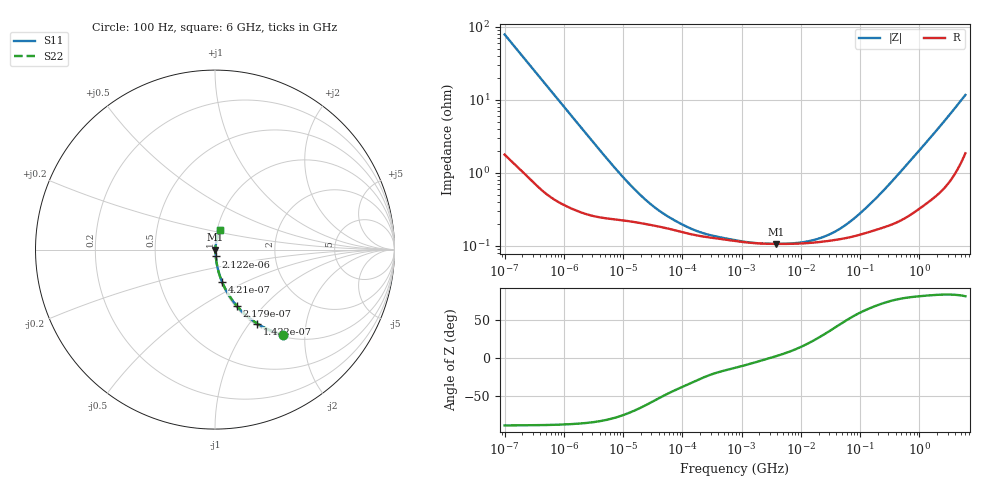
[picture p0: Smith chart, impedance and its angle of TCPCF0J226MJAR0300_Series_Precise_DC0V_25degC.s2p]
! TCPCF0J226MJAR0300 Polymer Tantalum Capacitor Sparameter Model
! Model Generated by Samsung Electro-Mechanics
! Samsung Sparameter Version 5.0
! Date : Oct-10-2024
! Products : Polymer Tantalum Capacitor
! Characteristics :
!  Nominal Capacitance = 22uF
!  Capacitance Tolerance = +/-20%
!  ESR = 300 mohm max at 100kHz
!  Rated Voltage = 6.3Vdc
!  Size = 0603(unit:inch), 1608(unit:mm)
!  Length = 1.60+/-0.20mm
!  Width = 0.80+/-0.20mm
!  Thickness = 0.90+/-0.10mm
!  Lineup = Conductive Polymer Type
!  Feature = PCF
!  Measurement Temperature : 25degC.
!  DC bias Value = 0V
!  Frequency : 100Hz ~ 6GHz
! External Node Assignments :
!  1  o---||---o  2
# MHz S RI R 50.0
! Freq.  Real(S11)  Im(S11)  Real(S12)  Im(S12)  Real(S21)  Im(S21)  Real(S22)  Im(S22)
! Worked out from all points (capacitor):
!   300 points, 100 Hz to 6 GHz, reference 50 ohm
!   read as one part in series: C = 20.4 uF near 106.2 Hz
!   lowest |Z| = 106 mohm at 3.788 MHz (marker M1)
!   series resonance near 3.084 MHz, so ESL is about 130 pH
!   S11 on the Smith chart (normalised r, x): 100 Hz: 1.04, -1.56; 143.2 Hz: 1.03, -1.09; 217.9 Hz: 1.02, -0.72; 421 Hz: 1.01, -0.38; 2.122 kHz: 1.01, -0.08; 6 GHz: 1.04, +0.23
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0.0001  0.3803 -0.4742  0.6197 0.4742  0.6197 0.4742  0.3803 -0.4742
0.0001432463  0.2353 -0.4121  0.7647 0.4121  0.7647 0.4121  0.2353 -0.4121
0.0002178615  0.122 -0.3142  0.878 0.3142  0.878 0.3142  0.122 -0.3142
0.0004210496  0.0396 -0.1802  0.9604 0.1802  0.9604 0.1802  0.0396 -0.1802
0.0008639723  0.0123 -0.0912  0.9877 0.0912  0.9877 0.0912  0.0123 -0.0912
0.001998454  0.00446 -0.0402  0.9955 0.0402  0.9955 0.0402  0.00446 -0.0402
0.002121818  0.00423 -0.0379  0.9958 0.0379  0.9958 0.0379  0.00423 -0.0379
0.01205343  0.00223 -0.00701  0.9978 0.00701  0.9978 0.00701  0.00223 -0.00701
0.02194065  0.00203 -0.00406  0.998 0.00406  0.998 0.00406  0.00203 -0.00406
0.03993819  0.00184 -0.00243  0.9982 0.00243  0.9982 0.00243  0.00184 -0.00243
0.08195114  0.0016 -0.0014  0.9984 0.0014  0.9984 0.0014  0.0016 -0.0014
0.1681596  0.0014 -0.00081  0.9986 0.00081  0.9986 0.00081  0.0014 -0.00081
0.7981464  0.00116 -0.000265  0.9988 0.000265  0.9988 0.000265  0.00116 -0.000265
3.788293  0.00106 3.89e-05  0.9989 -3.89e-05  0.9989 -3.89e-05  0.00106 3.89e-05
8.253232  0.00107 0.000216  0.9989 -0.000216  0.9989 -0.000216  0.00107 0.000216
15.95059  0.0011 0.000449  0.9989 -0.000449  0.9989 -0.000449  0.0011 0.000449
30.82687  0.00117 0.000831  0.9988 -0.000831  0.9988 -0.000831  0.00117 0.000831
59.57749  0.00128 0.0015  0.9987 -0.0015  0.9987 -0.0015  0.00128 0.0015
129.7964  0.00152 0.00301  0.9985 -0.00301  0.9985 -0.00301  0.00152 0.00301
318.7652  0.00195 0.0068  0.998 -0.0068  0.998 -0.0068  0.00195 0.0068
1922.593  0.00613 0.0366  0.9939 -0.0366  0.9939 -0.0366  0.00613 0.0366
6000  0.0304 0.109  0.9696 -0.109  0.9696 -0.109  0.0304 0.109
